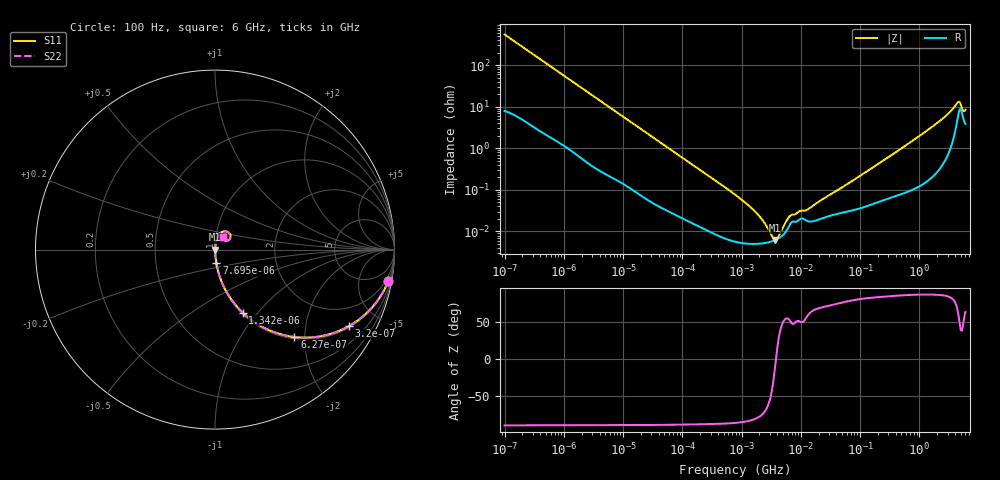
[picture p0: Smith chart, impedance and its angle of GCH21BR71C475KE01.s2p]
!Murata Part Number: GCH21BR71C475KE01
!These Parameters are Measured in Series Mode Connection
!Data Generated on Mar 13, 2026
!  o--ll--o
!Port1  Port2
!  o------o
!Operation Temp=25[degC], DC Bias Voltage=0[V]
!Freq. Start=100[Hz] Stop=6[GHz] 401[Steps]
# Hz S RI R 50
!Freq.(Hz) S11(Real) S11(Imag) S21(Real) S21(Imag) S12(Real) S12(Imag) S22(Real) S22(Imag)
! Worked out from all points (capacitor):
!   401 points, 100 Hz to 6 GHz, reference 50 ohm
!   read as one part in series: C = 2.91 uF near 109 Hz
!   lowest |Z| = 6.26 mohm at 3.712 MHz (marker M1)
!   series resonance near 3.804 MHz, so ESL is about 600 pH
!   S11 on the Smith chart (normalised r, x): 100 Hz: 1, -11; 320 Hz: 1.06, -3.45; 627 Hz: 1.03, -1.78; 1.342 kHz: 1.02, -0.84; 7.695 kHz: 1.00, -0.15; 6 GHz: 1.08, +0.15
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100  0.9649 -0.1768  0.0351 0.1768  0.0351 0.1768  0.9649 -0.1768
196  0.8829 -0.3128  0.1171 0.3128  0.1171 0.3128  0.8829 -0.3128
320  0.7445 -0.4272  0.2555 0.4272  0.2555 0.4272  0.7445 -0.4272
627  0.442 -0.4869  0.558 0.4869  0.558 0.4869  0.442 -0.4869
1342  0.1546 -0.3514  0.8454 0.3514  0.8454 0.3514  0.1546 -0.3514
2008  0.0779 -0.2583  0.9221 0.2583  0.9221 0.2583  0.0779 -0.2583
7695  0.00724 -0.074  0.9928 0.074  0.9928 0.074  0.00724 -0.074
40335  0.00061 -0.0146  0.9994 0.0146  0.9994 0.0146  0.00061 -0.0146
774597  5.73e-05 -0.000769  0.9999 0.000769  0.9999 0.000769  5.73e-05 -0.000769
1734173  5.03e-05 -0.000286  0.9999 0.000286  0.9999 0.000286  5.03e-05 -0.000286
2967816  5.57e-05 -8.33e-05  0.9999 8.33e-05  0.9999 8.33e-05  5.57e-05 -8.33e-05
3712478  6.21e-05 -8.1e-06  0.9999 8.1e-06  0.9999 8.1e-06  6.21e-05 -8.1e-06
4643984  7.5e-05 6.88e-05  0.9999 -6.88e-05  0.9999 -6.88e-05  7.5e-05 6.88e-05
6644369  0.000152 0.000186  0.9998 -0.000186  0.9998 -0.000186  0.000152 0.000186
9506416  0.000195 0.000237  0.9998 -0.000237  0.9998 -0.000237  0.000195 0.000237
1.243624e7  0.000182 0.000269  0.9998 -0.000269  0.9998 -0.000269  0.000182 0.000269
1.555665e7  0.000175 0.000364  0.9998 -0.000364  0.9998 -0.000364  0.000175 0.000364
3.124326e8  0.000669 0.00629  0.9993 -0.00629  0.9993 -0.00629  0.000669 0.00629
1.95892e9  0.00412 0.0392  0.9959 -0.0392  0.9959 -0.0392  0.00412 0.0392
4.385646e9  0.057 0.1025  0.943 -0.1025  0.943 -0.1025  0.057 0.1025
4.796499e9  0.087 0.0812  0.913 -0.0812  0.913 -0.0812  0.087 0.0812
6e9  0.0418 0.0694  0.9582 -0.0694  0.9582 -0.0694  0.0418 0.0694
